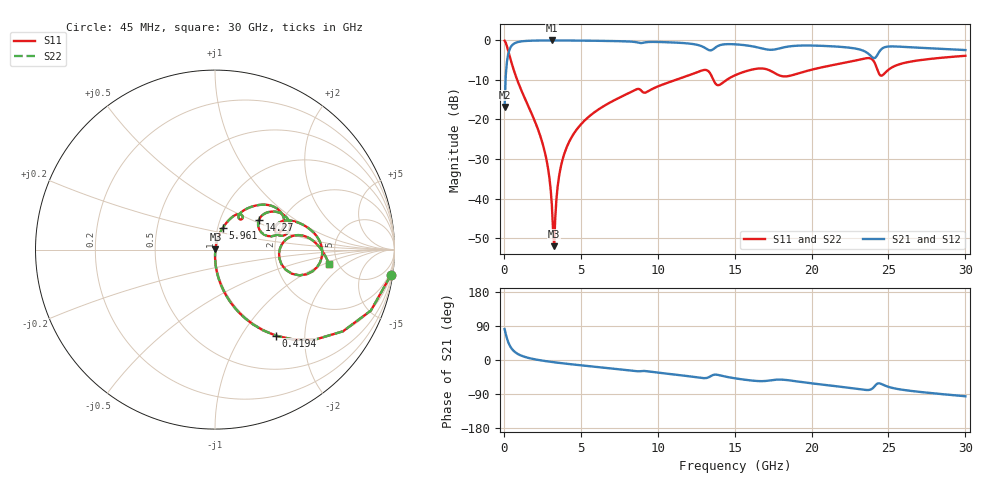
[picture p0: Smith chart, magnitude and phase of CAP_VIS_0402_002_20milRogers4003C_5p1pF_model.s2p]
! S-parameter model data by Modelithics Inc.  support@modelithics.com  813-866-6335  Tampa FL USA
! S-Parameter data specifications:
! Substrate: 20-mil Rogers 4003C, substrate thickness, H=0.508mm, Dielectric constant, Er=3.75
! PCB Mounting Pad Footprint: Pad width, PadW=0.50mm , Pad length, PadL=0.50mm , Pad gap, PadG (edge-to-edge)=0.40mm , Reference planes=1.4mm apart
! Created Wed Nov 18 12:48:07 2015
# hz S ma R 50
! 2 Port Network Data from SP1.SP block
! freq  magS11  angS11  magS21  angS21  magS12  angS12  magS22  angS22
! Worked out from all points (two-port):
!   401 points, 45 MHz to 30 GHz, reference 50 ohm
!   highest |S21| = -0.02 dB at 3.115 GHz (marker M1); lowest = -16.9 dB at 45 MHz (marker M2)
!   |S21| within 3 dB of the highest: 311.5 MHz to 23.57 GHz (23.26 GHz wide, 195 % of centre); 24.38 GHz to end of sweep
!   lowest |S11| = -52.0 dB at 3.265 GHz (marker M3), VSWR 1.01, Z = 50.2 + j0.071 ohm
!   |S11| at or under -10 dB: 864.4 MHz to 11.18 GHz (10.31 GHz wide, 171 % of centre); 13.62 GHz to 14.48 GHz (857.1 MHz wide, 6.1 % of centre)
!   |S22| runs from -52.0 to -0.1 dB; largest |S21 - S12| = 0
!   S11 on the Smith chart (normalised r, x): 45 MHz: 1, -14; 419.4 MHz: 0.98, -1.44; 5.961 GHz: 1.06, +0.26; 14.27 GHz: 1.53, +0.56; 30 GHz: 4.23, -1.11
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4.5e7  0.9896 -8.3  0.1436 81.7  0.1436 81.7  0.9896 -8.3
4.194375e8  0.5879 -54.7  0.8082 35.2  0.8082 35.2  0.5879 -54.7
1.018538e9  0.2647 -76.2  0.963 13.5  0.963 13.5  0.2647 -76.2
2.516288e9  0.0495 -89.4  0.9967 -1.7  0.9967 -1.7  0.0495 -89.4
2.890725e9  0.02259 -88.4  0.9975 -4.0  0.9975 -4.0  0.02259 -88.4
3.115388e9  0.008387 -79.6  0.9976 -5.2  0.9976 -5.2  0.008387 -79.6
3.265162e9  0.002503 16.4  0.9976 -6.0  0.9976 -6.0  0.002503 16.4
3.864262e9  0.03374 76.8  0.9968 -8.9  0.9968 -8.9  0.03374 76.8
5.062462e9  0.08916 73.8  0.9929 -14.3  0.9929 -14.3  0.08916 73.8
5.961112e9  0.1264 70.4  0.9885 -18.1  0.9885 -18.1  0.1264 70.4
1.007992e10  0.2652 54.2  0.954 -33.6  0.954 -33.6  0.2652 54.2
1.300054e10  0.4221 29.5  0.8184 -47.9  0.8184 -47.9  0.4221 29.5
1.359964e10  0.3225 13.2  0.771 -39.6  0.771 -39.6  0.3225 13.2
1.427362e10  0.296 34.1  0.8893 -42.6  0.8893 -42.6  0.296 34.1
1.50225e10  0.362 35.2  0.8916 -48.4  0.8916 -48.4  0.362 35.2
1.764356e10  0.3817 11.6  0.7701 -52.1  0.7701 -52.1  0.3817 11.6
2.003996e10  0.4275 22.3  0.8599 -61.7  0.8599 -61.7  0.4275 22.3
2.355968e10  0.5951 1.0  0.7077 -79.2  0.7077 -79.2  0.5951 1.0
2.415878e10  0.4913 -17.0  0.6069 -66.3  0.6069 -66.3  0.4913 -17.0
2.453321e10  0.3576 -3.0  0.7721 -63.2  0.7721 -63.2  0.3576 -3.0
2.505742e10  0.4338 9.9  0.8377 -71.6  0.8377 -71.6  0.4338 9.9
3e10  0.6385 -7.0  0.7542 -95.7  0.7542 -95.7  0.6385 -7.0
